// Module to select via sensor, cylinder and axis
FUNCTION_BLOCK FB_SortingModule EXTENDS FB_Subsystem_Root
VAR_INPUT
	// =============== Cylinder buttons =============================================
	bButtonCylToWorkIn	AT%I*	: BOOL;							// Signal of button to move cylinder to work position
	bButtonCylToBaseIn			: BOOL;							// Signal of button to move cylinder to base position
END_VAR
VAR_OUTPUT
	// =============== Process information ==========================================
	bSelected					: BOOL;							// Gets true if one sorting process is done
	
	// =============== For movement simulation on visualization =====================
	bCylinderToWork				: BOOL;							// Simulation of cylinder movement to work position
	
	// =============== Error variables ==============================================
	bCylError					: BOOL;							// Error signal of cylinder
	sCylErrorMsg				: STRING;						// Error message of cylinder
	
	// =============== Temperature recording ========================================
	aTemps						: ARRAY[1..100] OF LREAL;		// Array with recorded temperatures of cylinder
	
	// =============== Button return signals ========================================
	bButtonCylToWorkOut			: BOOL;							// Processed signal for button to move cylinder to work position
	bButtonCylToBaseOut			: BOOL;							// Processed signal for button to move cylinder to base position
END_VAR
VAR
	// =============== Function block instance of sensor ============================	
	fbSensorDelay				: FB_SignalHandlingDelay;		// Sensor needed for sorting process
	
	// =============== Function block instances for cylinder ========================
	fbCylinder					: FB_Cylinder;					// Without diagnosis and temperature mode
	//fbCylinderDiag				: FB_CylinderDiag;				// With diagnosis of states
	//fbCylinderTemp				: FB_CylinderTemp;				// With temperature mode
	//fbCylinderTempDiag			: FB_CylinderTempDiag;			// With diagnosis of temperature
	//fbCylinderTempRecord		: FB_CylinderTempRecord;		// With record of temperatures
	
	// =============== Interface instance for cylinder ==============================
	//fbCylinder					: I_Cylinder;					// Interface for flexible access to cylinder FBs
	
	// =============== Submodule parameters =========================================
	tTimeOutCylinder			: TIME;							// For cylinder with diagnosis: time in which the cylinder should reach base/work position
	tRecordIntervalCylinder		: TIME;							// Time of intervals to record the temperature of cylinder
	tSensorDelay				: TIME;							// Time to delay sensor signal (time between hardware and processed software signal)
	tMoveAxis					: TIME;							// Time to move axis
	
	// =============== Manual cylinder control ======================================
	fbButtonCylToWork			: FB_SignalHandling	;	// To move cylinder manually to work position
	fbButtonCylToBase			: FB_SignalHandling;		// To move cylinder manually to base position

	// =============== Common variables =============================================
	fbTimerAxis					: TON;							// Timer to move axis in (semi) automatic mode	
	fbTriggerCylAtWork			: R_TRIG;						// Trigger to recognize rising edge of cylinder being at work position
	eStateAutoAxis				: E_StateSortingAutoAxis;		// State variable for automatic mode - process to move axis
	eStateAutoCylinder			: E_StateSortingAutoCylinder;	// State variable for automatic mode - process to move cylinder
	
	_ObjectName					: STRING := 'FB_SortingModule';
END_VAR

// =========================================================
;
// =========================================================

METHOD Automatic
VAR_INPUT
END_VAR

VAR
	Stop: INT;
	bHalt: INT;
END_VAR
// =========================================================
// Process of sorting boxes - axis movement

	fbTriggerCylAtWork(CLK := fbCylinder.bState_AtWorkPos);			// Accessing property of FB via interface instance

	CASE eStateAutoAxis OF
		
		// =========================================================
		E_StateSortingAutoAxis.WaitForCylinderAtWorkPos:
		
						IF fbTriggerCylAtWork.Q THEN
							fbTimerAxis(IN := TRUE,
										PT := tMoveAxis);
										
							eStateAutoAxis := E_StateSortingAutoAxis.MoveAxis;
						END_IF
		
		// =========================================================
		E_StateSortingAutoAxis.MoveAxis:
		
						fbTimerAxis();
						
						IF bHaltRequest THEN
							eStateAutoAxis := E_StateSortingAutoAxis.StopAxis;
						ELSIF fbTimerAxis.Q THEN
							fbTimerAxis(IN := FALSE);
							
							bSelected 		:= TRUE;
							eStateAutoAxis	:= E_StateSortingAutoAxis.StopAxis;
						ELSE
							fbAxis.MoveFw();
						END_IF
		
		
		// =========================================================
		E_StateSortingAutoAxis.StopAxis:
		
						bSelected := FALSE;
						
						IF NOT bHaltDone THEN
							Halt(bHalt := TRUE);
						ELSE
							Halt(bHalt := FALSE);
							
							eStateAutoAxis := E_StateSortingAutoAxis.WaitForCylinderAtWorkPos;
						END_IF
						
(*   可不可以将以上代码改为以下呢：

						Halt(bHalt := NOT bHaltDone);
						
						IF  bHaltDone THEN	
							eStateAutoAxis := E_StateSortingAutoAxis.WaitForCylinderAtWorkPos;
						END_IF
						
                         答案：不可以，否则HaltDone无法复位 *)
						
	END_CASE
	
// =========================================================
// Process of sorting boxes - cylinder movement

	CASE eStateAutoCylinder OF
		
		// =========================================================
		// Detecting a box
		E_StateSortingAutoCylinder.DetectBox:	
		
					fbCylinder.MoveToBase();								// Calling method of FB via interface instance
					
					IF fbSensorDelay.bOut THEN
						eStateAutoCylinder := E_StateSortingAutoCylinder.CylToWork;
					END_IF
			
		// =========================================================
		// Moving cylinder to work position
		E_StateSortingAutoCylinder.CylToWork:
		
					fbCylinder.MoveToWork();								// Calling method of FB via interface instance
					
					IF fbCylinder.bState_AtWorkPos THEN					// Accessing property of FB via interface instance
						eStateAutoCylinder := E_StateSortingAutoCylinder.CylToBase;
					END_IF
		
		// =========================================================
		// Moving cylinder back to base position
		E_StateSortingAutoCylinder.CylToBase:
		
					fbCylinder.MoveToBase();								// Calling method of FB via interface instance
					
					IF fbCylinder.bState_AtBasePos THEN					// Accessing property of FB via interface instance
						eStateAutoCylinder := E_StateSortingAutoCylinder.DetectBox;
					END_IF
	END_CASE

// =========================================================
END_METHOD

PROPERTY bState_CylinderAtBasePos : BOOL
GET
bState_CylinderAtBasePos := fbCylinder.bState_AtBasePos;
END_GET
END_PROPERTY

PROPERTY bState_CylinderAtWorkPos : BOOL
GET
bState_CylinderAtWorkPos := fbCylinder.bState_AtWorkPos;
END_GET
END_PROPERTY

METHOD CylinderOptions
VAR_INPUT
	bCylinderDiag		: BOOL;		// If true the cylinder has diagnosis functionality
	bCylinderTemp		: BOOL;		// IF true the cylinder has temperature functionality
	bCylinderRecord		: BOOL;		// If true the cylinder has recording functionality
END_VAR
// =========================================================
// Selecting cylinder

	// Checking variables to enable/disable diagnosis and temperature mode
	IF bCylinderDiag THEN
		IF bCylinderTemp THEN
			// ============== FB with diagnosis and temperature mode ==============
			bCylError 		:= fbCylinderTempDiag.bError;						// Assigning output variable of chosen FB to local output variable
			sCylErrorMsg 	:= fbCylinderTempDiag.sErrorMsg;
			fbCylinder		:= fbCylinderTempDiag;								// Assigning chosen FB instance to interface instance
		
		ELSE
			// ============== FB with diagnosis and without temperature mode ==============
			fbCylinderDiag.tTimeOut 	:= tTimeOutCylinder;					// Setting special data for selected FB
			bCylError 					:= fbCylinderDiag.bError;				// Assigning output variable of chosen FB to local output variable
			sCylErrorMsg 				:= fbCylinderDiag.sErrorMsg;		
			fbCylinder					:= fbCylinderDiag;						// Assigning chosen FB instance to interface instance
		END_IF
		
	ELSE
		bCylError 		:= FALSE;
		sCylErrorMsg 	:= '';
		
		IF bCylinderTemp THEN
			IF bCylinderRecord THEN
				// ============== FB without diagnosis and with temperature recording ==============
				fbCylinderTempRecord.tIntervalTime	:= tRecordIntervalCylinder;	// Time of record interval
				fbCylinderTempRecord.bRecordStart 	:= bComprAirEnabledLocal;	// Recording if compressed air is set
				
				fbCylinderTempRecord.Record();									// Calling method of function block FB_CylinderTempRecord
				
				aTemps		:= fbCylinderTempRecord.aTemps;						// Saving output variable
				fbCylinder 	:= fbCylinderTempRecord;							// Assigning chosen FB instance to interface instance
			ELSE
				// ============== FB without diagnosis and with temperature mode, but without recording ==============
				fbCylinder 	:= fbCylinderTemp; 									// Assigning chosen FB instance to interface instance
			END_IF
			
		ELSE
			// ============== FB without diagnosis and without temperature mode ==============
			fbCylinder := fbCylinder;											// Assigning chosen FB instance to interface instance					
		END_IF	
	END_IF
									
// =========================================================
END_METHOD

METHOD Enable
VAR_INPUT
	bComprAirEnabled		: BOOL;			// Enable of compressed air
	bAxisEnable				: BOOL;			// Enable of axis
	bSensorEnable			: BOOL;			// Enable of sensor
	bManualAxisEnable		: BOOL;			// Enable of manual axis control
END_VAR
// =========================================================
// Calling method Enable of base class FB_Module via 'SUPER^.'
		
	SUPER^.Enable(	bComprAirEnabled	:= bComprAirEnabled,
					bAxisEnable			:= bAxisEnable,
					bSensorEnable		:= bSensorEnable,
					bManualAxisEnable	:= bManualAxisEnable);

// =========================================================
// Sensor control
		
	fbSensorDelay.Enable(bEnable := bSensorEnable);

// =========================================================
// Cylinder control (accessing property of FB via interfaces intance)
		
	fbButtonCylToWork.Enable( bEnable := bManualCylinderEnable );
	fbButtonCylToBase.Enable( bEnable := bManualCylinderEnable );


// =========================================================
END_METHOD

METHOD InputOutput
VAR_INPUT
END_VAR
// =========================================================
// Calling method SetOutput of base class FB_Module via 'SUPER^.'
		
	SUPER^.InputOutput();

// =========================================================
// Sensor
		
	fbSensorDelay.SetOutput();

// =========================================================
// Cylinder buttons
		
	fbButtonCylToWork.SetOutput();
	fbButtonCylToBase.SetOutput();

// =========================================================
// Output variables for cylinder
		
	bCylinderToWork := fbCylinder.bState_MoveToWork;		// Accessing property of selected FB via interface instance

// =========================================================
// Buttons
    bButtonCylToBaseIn:= NOT bButtonCylToWorkIn;
	fbButtonCylToBase( bInput:= bButtonCylToBaseIn AND NOT bButtonCylToWorkIn , bOut=>bButtonCylToBaseOut );
	fbButtonCylToWork( bInput:= bButtonCylToWorkIn AND NOT bButtonCylToBaseIn, bOut=>bButtonCylToWorkOut );
	
// =========================================================
END_METHOD

METHOD Maintenance
VAR_INPUT
END_VAR
// =========================================================
// Calling own method Manual of this class FB_SortingModule via 'THIS^.'
		
	THIS^.Manual();

// =========================================================
END_METHOD

METHOD Manual
VAR_INPUT
END_VAR
// =========================================================
// Calling method Manual of base class FB_Module via 'SUPER^.'
		
	SUPER^.Manual();

// =========================================================
// Manual cylinder control (Calling methods of FB via interface instance)
	
	// Cylinder to work position
	IF fbButtonCylToWork.bOut THEN
		fbCylinder.MoveToWork();
	// Cylinder to base position
	ELSIF fbButtonCylToBase.bOut THEN
		fbCylinder.MoveToBase();
	END_IF

// =========================================================
END_METHOD

METHOD Reset
VAR_INPUT
	bReset		: BOOL;				// True if machine is in state RESETTING
END_VAR
// =========================================================
// Calling action Reset of base class FB_Module via 'SUPER^.'
		
	SUPER^.Reset(bReset := bReset);

// =========================================================
// Resetting cylinder and axis
	
	IF fbTriggerResetStart.Q THEN
		bSelected := FALSE;
		
		fbTimerAxis(IN := FALSE);
		
		// Calling method of FB via interface instance
		fbCylinder.Reset();
	END_IF

// =========================================================
END_METHOD

METHOD PROTECTED ResetState
VAR_INPUT
END_VAR
// =========================================================

eStateAutoAxis		:= E_StateSortingAutoAxis.WaitForCylinderAtWorkPos;
eStateAutoCylinder 	:= E_StateSortingAutoCylinder.DetectBox;

// =========================================================
END_METHOD

METHOD Semiautomatic
VAR_INPUT
END_VAR
// =========================================================
// Calling own method Automatic of this class FB_SortingModule via 'THIS^.'
		
	THIS^.Automatic();				

// =========================================================
END_METHOD

METHOD Starting
VAR_INPUT
	bStarting		: BOOL;			// True if machine is in state STARTING
END_VAR
// =========================================================
// Setting time to delay sensor
		
	fbSensorDelay.tDelay := tSensorDelay;

// =========================================================
// Calling method Starting of base class FB_Module via 'SUPER^.'
		
	SUPER^.Starting(bStarting := bStarting);

// =========================================================
END_METHOD

PROPERTY tAxisMovement : TIME
GET
tAxisMovement := tMoveAxis;
END_GET
SET
tMoveAxis := tAxisMovement;
END_SET
END_PROPERTY

PROPERTY tDelayOfSensor : TIME
GET
tDelayOfSensor := tSensorDelay;
END_GET
SET
tSensorDelay := tDelayOfSensor;
END_SET
END_PROPERTY

PROPERTY tRecordIntervalOfCylinder : TIME
GET
tRecordIntervalOfCylinder := tRecordIntervalCylinder;
END_GET
SET
tRecordIntervalCylinder := tRecordIntervalOfCylinder;
END_SET
END_PROPERTY

PROPERTY tTimeOutOfCylinder : TIME
GET
tTimeOutOfCylinder := tTimeOutCylinder;
END_GET
SET
tTimeOutCylinder := tTimeOutOfCylinder;
END_SET
END_PROPERTY

END_FUNCTION_BLOCK
